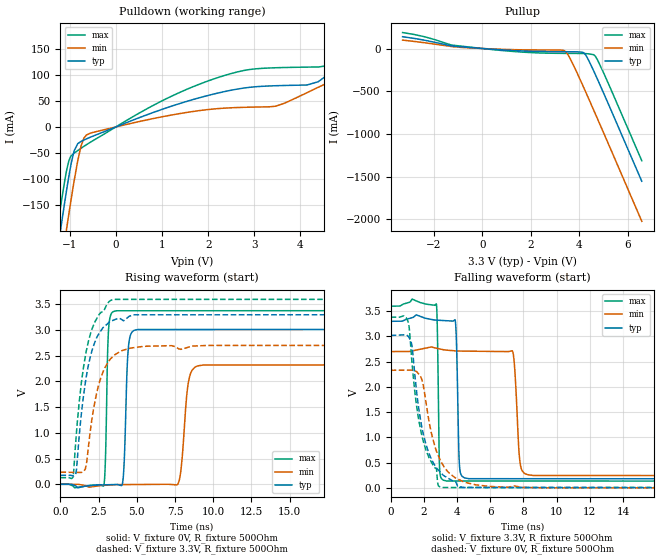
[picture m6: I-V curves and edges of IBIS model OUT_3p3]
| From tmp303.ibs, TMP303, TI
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|   Model
[Model]   OUT_3p3
Model_type   Output
Polarity   Non-Inverting
Vmeas = 1.65
Vref = 0
Cref = 1pF
Rref = 100000
|   typ   min   max
C_comp   1pF   1pF   1pF
[Voltage Range]   3.3   2.7   3.6
[Temperature Range]   25   125   -40
[Pullup Reference]   3.3   2.7   3.6
[Pulldown Reference]   -0   -0   -0
[Power Clamp Reference]   3.3   2.7   3.6
[GND Clamp Reference]   -0   -0   -0
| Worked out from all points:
|   slope of the pulldown table from 0 to 0.495 V, typ, clamps not added: 28.4 ohm
|   slope of the pullup table from 0 to 0.495 V, typ, clamps not added: 47.9 ohm
|   falling waveform, V_fixture 3.3V, R_fixture 500Ohm: 20-80 % time 121ps typ, 225ps min, 88.7ps max; typ from 3.3 V to 0.174 V
|   rising waveform, V_fixture 0V, R_fixture 500Ohm: 20-80 % time 194ps typ, 366ps min, 140ps max; typ from 0 V to 3.02 V
|   rising waveform, V_fixture 3.3V, R_fixture 500Ohm: 20-80 % time 953ps typ, 985ps min, 945ps max; typ from 0.174 V to 3.3 V
|   falling waveform, V_fixture 0V, R_fixture 500Ohm: 20-80 % time 1ns typ, 1.08ns min, 983ps max; typ from 3.02 V to 0 V
[Pulldown]
|   Voltage   I(typ)   I(min)   I(max)
-3.3V     -1.561A    -1.634A    -1.518A
-1.27V    -242.4mA   -319.8mA   -197mA
-1.211V   -206.1mA   -283.2mA   -161.4mA
-1.063V   -119.3mA   -193.6mA   -81.84mA
-904.2mV  -46.16mA   -104.1mA   -50.42mA
-755.7mV  -28mA      -37.35mA   -41.17mA
-547.8mV  -19.62mA   -11.89mA   -29.17mA
1.69V     53.14mA    29.94mA    77.98mA
3.472V    79.29mA    40.1mA     113.9mA
4.759V    111.6mA    91.74mA    120mA
5.392V    153.7mA    116.3mA    185.5mA
6.59V     216.7mA    156mA      282.4mA
[Pullup]
|   Voltage   I(typ)   I(min)   I(max)
-3.3V     138mA      98.29mA    186.6mA
-2.419V   98.31mA    68.51mA    139.2mA
-1.181V   27.03mA    20.12mA    37.34mA
1.393V    -25.49mA   -14.13mA   -37.05mA
3.204V    -37.34mA   -18.15mA   -56.41mA
3.432V    -37.77mA   -33.99mA   -56.95mA
3.699V    -38.2mA    -157.7mA   -57.44mA
4.224V    -58.94mA   -479.5mA   -58.71mA
4.382V    -132.4mA   -580.5mA   -62.59mA
4.67V     -304.7mA   -765.3mA   -90.6mA
5.056V    -550.6mA   -1.016A    -313.1mA
6.59V     -1.555A    -2.023A    -1.314A
[Ramp]
R_load = 500
|   typ   min   max
dV/dt_r   1.81109/1.94072e-10   1.39771/3.66049e-10   2.02927/1.39708e-10
dV/dt_f   1.87564/1.20684e-10   1.47868/2.25316e-10   2.0831/8.87333e-11
[Falling Waveform]
V_fixture = 3.3V
V_fixture_min = 2.7V
V_fixture_max = 3.6V
R_fixture = 500Ohm
C_fixture = 0F
|   Time   V(typ)   V(min)   V(max)
0s        3.3V       2.7V       3.6V
2.747ns   3.323V     2.767V     3.648V
2.951ns   3.319V     2.752V     370mV
3.386ns   3.311V     2.729V     135.5mV
3.906ns   3.287V     2.713V     135.4mV
4.71ns    181.5mV    2.708V     135.4mV
7.33ns    181.3mV    2.716V     135.2mV
7.794ns   181.2mV    498.1mV    135.1mV
8.609ns   181.2mV    244.5mV    135.1mV
100ns     173.9mV    235.5mV    128.2mV
[Rising Waveform]
V_fixture = 0V
V_fixture_min = 0V
V_fixture_max = 0V
R_fixture = 500Ohm
C_fixture = 0F
|   Time   V(typ)   V(min)   V(max)
0s        818.9pV    2.374nV    587.1pV
2.828ns   -11.53mV   -20.43mV   -28.47mV
3.151ns   -8.551mV   -15.63mV   3.02V
3.639ns   -4.064mV   -8.384mV   3.374V
4.468ns   2.721V     -5.596mV   3.374V
5.051ns   3.009V     -4.308mV   3.374V
7.69ns    3.009V     6.541mV    3.374V
8.442ns   3.009V     2.083V     3.374V
9.366ns   3.009V     2.319V     3.374V
100ns     3.018V     2.33V      3.382V
[Rising Waveform]
V_fixture = 3.3V
V_fixture_min = 2.7V
V_fixture_max = 3.6V
R_fixture = 500Ohm
C_fixture = 0F
|   Time   V(typ)   V(min)   V(max)
0s        173.9mV    235.5mV    128.2mV
842.5ps   161.8mV    232.2mV    172mV
1.047ns   278.8mV    231.4mV    998.8mV
1.328ns   1.255V     230.3mV    1.864V
1.628ns   1.974V     295.6mV    2.488V
2.106ns   2.64V      1.356V     3.049V
2.46ns    2.9V       1.886V     3.264V
3.497ns   3.194V     2.501V     3.595V
7.237ns   3.295V     2.695V     3.595V
100ns     3.3V       2.7V       3.6V
[Falling Waveform]
|Gnd
V_fixture = 0V
V_fixture_min = 0V
V_fixture_max = 0V
R_fixture = 500Ohm
C_fixture = 0F
|   Time   V(typ)   V(min)   V(max)
0s        3.018V     2.33V      3.382V
1.051ns   3.003V     2.332V     3.294V
1.281ns   2.818V     2.333V     2.501V
1.833ns   1.285V     2.184V     1.107V
2.46ns    566.6mV    1.076V     505.7mV
2.863ns   357.4mV    646mV      50.68mV
3.172ns   250mV      440.5mV    7.245mV
5.124ns   7.178mV    59.73mV    7.099mV
9.424ns   6.853mV    183.9uV    6.777mV
100ns     818.9pV    2.374nV    625.9pV
